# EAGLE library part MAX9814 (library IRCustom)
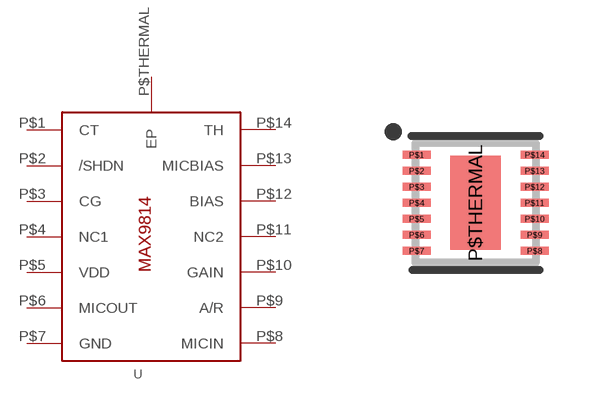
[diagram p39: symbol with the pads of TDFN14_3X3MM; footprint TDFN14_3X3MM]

Designator prefix -

## MAX9814TDFN14  [TDFN14_3X3MM]
P$1  CT
P$2  /SHDN
P$3  CG
P$4  NC1  nc
P$5  VDD
P$6  MICOUT
P$7  GND
P$8  MICIN
P$9  A/R
P$10  GAIN
P$11  NC2  nc
P$12  BIAS
P$13  MICBIAS
P$14  TH
P$THERMAL  EP

## Footprint TDFN14_3X3MM (pad centres in mm)
TDFN 14 3x3x0.75mm Source: http://datasheets.maxim-ic.com/en/ds/MAX98306.pdf Based on recommendtions in: http://www.freescale.com/files/sensors/doc/data_sheet/MAG3110.pdf
smd 0.7 x 0.2: P$1 -1.475,1.2; P$2 -1.475,0.8; P$3 -1.475,0.4; P$4 -1.475,0; P$5 -1.475,-0.4; P$6 -1.475,-0.8; P$7 -1.475,-1.2; P$8 1.475,-1.2; P$9 1.475,-0.8; P$10 1.475,-0.4; P$11 1.475,0; P$12 1.475,0.4; P$13 1.475,0.8; P$14 1.475,1.2
smd 1.27 x 2.35: P$THERMAL 0,0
